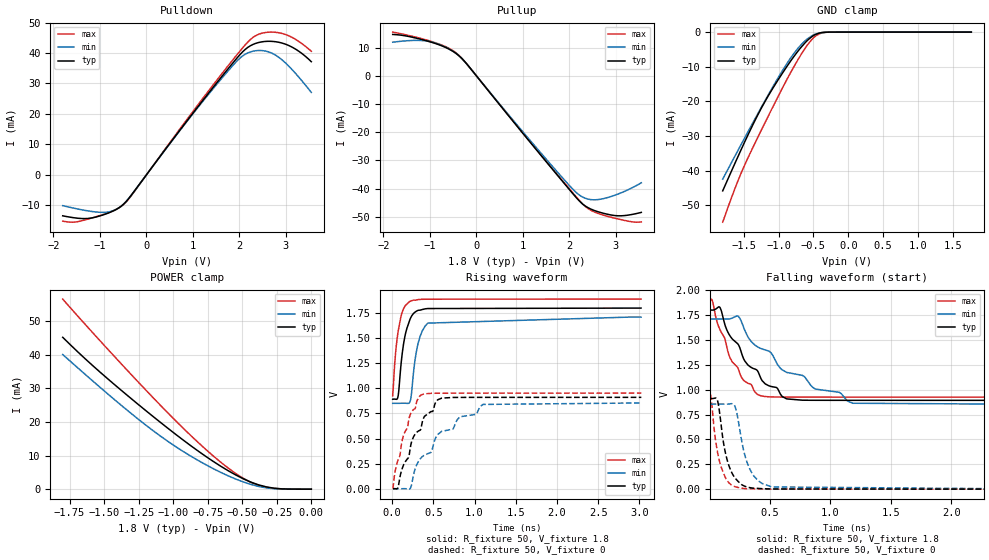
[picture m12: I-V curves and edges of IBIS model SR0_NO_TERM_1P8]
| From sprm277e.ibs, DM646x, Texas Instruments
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|   Model Cell SR0_NO_TERM_1P8
|Driver model in Slow Mode of operation, 1P8V +/-5% Operation
[Model]   SR0_NO_TERM_1P8
Model_type   I/O
Polarity   Non-Inverting
Enable   Active-Low
Cref =  15.0000pF
Rref =  100.0000M
Vref =  0V
Vmeas =  0.9
C_comp   1.4932869p   1.4443092p   1.7624819p
[Temperature Range]   25   125   -40
[Voltage Range]   1.8   1.71   1.89
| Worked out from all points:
|   slope of the pulldown table from 0 to 0.27 V, typ, clamps not added: 48.6 ohm
|   slope of the pullup table from 0 to 0.27 V, typ, clamps not added: 48.6 ohm
|   GND clamp passes 1 mA (typ) near -0.50 V on its own axis
|   POWER clamp passes 1 mA (typ) near -0.36 V on its own axis
|   rising waveform, R_fixture 50, V_fixture 1.8: 20-80 % time 96.8ps typ, 105ps min, 81.4ps max; typ from 0.892 V to 1.8 V
|   rising waveform, R_fixture 50, V_fixture 0: 20-80 % time 290ps typ, 516ps min, 193ps max; typ from 0 V to 0.911 V
|   falling waveform, R_fixture 50, V_fixture 1.8: 20-80 % time 310ps typ, 539ps min, 209ps max; typ from 1.8 V to 0.892 V
|   falling waveform, R_fixture 50, V_fixture 0: 20-80 % time 90.3ps typ, 108ps min, 79.5ps max; typ from 0.911 V to 0 V
[POWER_clamp]
|   voltage   I(typ)   I(min)   I(max)
-1.8V     45.24mA    40.11mA    56.63mA
-1.527V   34.78mA    30.26mA    44.1mA
-1.309V   27.14mA    22.71mA    34.37mA
-1.091V   19.85mA    15.77mA    24.92mA
-872.7mV  12.95mA    9.842mA    15.97mA
-709.1mV  8.24mA     6.092mA    9.863mA
-600mV    5.448mA    3.934mA    6.223mA
-490.9mV  3.058mA    2.131mA    3.184mA
-436.4mV  2.077mA    1.4mA      2.009mA
-327.3mV  690.5uA    396.8uA    556.8uA
-218.2mV  104.2uA    49.84uA    76.16uA
0V        110.7nA    133.6nA    263.4nA
[Pulldown]
|   voltage   I(typ)   I(min)   I(max)
-1.8V     -13.46mA   -10.11mA   -15.21mA
-1.2V     -14.22mA   -11.97mA   -14.28mA
-818.2mV  -12.54mA   -12.18mA   -12.43mA
-545.5mV  -10.33mA   -10.31mA   -10.38mA
-327.3mV  -6.717mA   -6.686mA   -6.887mA
1.473V    29.47mA    29.01mA    30.28mA
1.964V    38.65mA    37.65mA    39.75mA
2.182V    41.88mA    40.06mA    43.65mA
2.455V    43.6mA     40.84mA    46.39mA
2.782V    43.71mA    39.26mA    46.8mA
3.164V    41.67mA    34.04mA    44.88mA
3.545V    37.15mA    27.06mA    40.58mA
[Pullup]
|   voltage   I(typ)   I(min)   I(max)
-1.8V     14.69mA    11.94mA    15.53mA
-1.036V   12.27mA    12.26mA    12.54mA
-709.1mV  10.41mA    10.55mA    10.69mA
-436.4mV  7.93mA     7.944mA    8.142mA
-218.2mV  4.442mA    4.38mA     4.432mA
1.8V      -36.42mA   -35.22mA   -36.18mA
2.127V    -42.84mA   -41.11mA   -42.58mA
2.291V    -45.59mA   -43.06mA   -45.6mA
2.564V    -47.94mA   -43.97mA   -48.49mA
2.945V    -49.5mA    -42.54mA   -50.39mA
3.218V    -49.51mA   -40.74mA   -51.41mA
3.545V    -48.45mA   -37.94mA   -51.83mA
[GND_clamp]
|   voltage   I(typ)   I(min)   I(max)
-1.8V     -45.84mA   -42.45mA   -54.88mA
-1.655V   -39.23mA   -36.93mA   -46.76mA
-1.509V   -32.77mA   -31.45mA   -39.47mA
-1.327V   -25.11mA   -24.68mA   -31.64mA
-1.145V   -18.35mA   -18.07mA   -24.19mA
-927.3mV  -11.35mA   -10.59mA   -15.5mA
-781.8mV  -7.112mA   -6.235mA   -10.08mA
-636.4mV  -3.474mA   -2.848mA   -5.206mA
-490.9mV  -889.6uA   -748.3uA   -1.49mA
-381.8mV  -136uA     -148.6uA   -241.8uA
-272.7mV  -12.55uA   -20.62uA   -15.52uA
1.764V    38.35nA    927.7nA    122.5nA
[Ramp]
| variable   typ   min   max
dV/dt_f  0.5640347/0.31110235n 0.53394643/0.5442772n 0.59146656/0.21041989n
dV/dt_r 0.54760551/0.28336882n 0.51543066/0.51694685n 0.57392976/0.19376821n
R_load = 50
[Rising Waveform]
R_fixture = 50
V_fixture = 1.8
V_fixture_min = 1.71
V_fixture_max = 1.89
|   time   V(typ)   V(min)   V(max)
7.268ps   892.3mV    851.1mV    924.5mV
37.84ps   892.5mV    851.1mV    1.31V
69.46ps   911.3mV    851.1mV    1.547V
102.4ps   1.188V     851.5mV    1.695V
155.2ps   1.518V     852.3mV    1.818V
212.3ps   1.677V     858.7mV    1.864V
234.8ps   1.718V     947mV      1.873V
309ps     1.775V     1.426V     1.884V
433.9ps   1.796V     1.65V      1.889V
3.019ns   1.8V       1.71V      1.89V
[Rising Waveform]
R_fixture = 50
V_fixture = 0
V_fixture_min = 0
V_fixture_max = 0
|   time   V(typ)   V(min)   V(max)
10.84ps   42.55uV    30.99uV    50.39uV
69.86ps   10.71mV    6.023uV    280mV
135ps     229.2mV    206.8uV    522.5mV
222.1ps   414.5mV    5.665mV    741.8mV
290.2ps   554.8mV    222.3mV    834.8mV
366.9ps   667.5mV    319.9mV    939mV
471.2ps   768.9mV    361.9mV    950.6mV
601.9ps   902.6mV    571.7mV    951.9mV
1.102ns   910.3mV    839.9mV    952.4mV
3.023ns   910.7mV    854.5mV    952.8mV
[Falling Waveform]
R_fixture = 50
V_fixture = 1.8
V_fixture_min = 1.71
V_fixture_max = 1.89
|   time   V(typ)   V(min)   V(max)
7.268ps   1.8V       1.71V      1.89V
26.33ps   1.799V     1.71V      1.887V
87.64ps   1.824V     1.71V      1.602V
174.1ps   1.533V     1.713V     1.311V
239.5ps   1.452V     1.735V     1.206V
323.2ps   1.243V     1.521V     1.063V
425.4ps   1.113V     1.413V     938.5mV
639.3ps   907.2mV    1.173V     925.5mV
1.184ns   892.7mV    863.3mV    924.9mV
3.019ns   892.3mV    851.1mV    924.5mV
[Falling Waveform]
R_fixture = 50
V_fixture = 0
V_fixture_min = 0
V_fixture_max = 0
|   time   V(typ)   V(min)   V(max)
10.84ps   910.7mV    854.5mV    952.8mV
61.98ps   905.6mV    854.5mV    406.3mV
87.58ps   739.1mV    854.5mV    262.1mV
142.7ps   312.1mV    854.2mV    93.2mV
218.6ps   102.6mV    804.7mV    22.27mV
279.8ps   36.44mV    405.7mV    7.457mV
332.2ps   15.77mV    205.9mV    4.172mV
405.2ps   7.295mV    82.51mV    2.032mV
516.5ps   1.897mV    22.18mV    996.5uV
3.023ns   42.55uV    30.99uV    50.39uV
